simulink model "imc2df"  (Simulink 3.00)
settings: Solver=ode45  SolverMode=SingleTasking  StartTime=0.0  StopTime=10  FixedStep=st_size  MaxStep=st_size  RelTol=1e-5  AbsTol=1e-6
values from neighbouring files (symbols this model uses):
  d_through_p = get(MAIN_MENU(19),'Value')    [cback.m]    (also in imcmenu.m = 0)
  Disturb = Setpoint    [mimo_MSF1DF_sim.m]    (also in mimo_MSF2DF_sim.m)
  Satlb = temp1    [cback.m]    (also in imcmenu.m = str2num(satlbs))
  Satub = temp1    [cback.m]    (also in imcmenu.m = str2num(satubs))
  Setpoint = zeros(1,n)    [mimo_MSF1DF_sim.m]    (also in mimo_MSF2DF_sim.m)
undefined symbols (not defined in the file or in its folder): denCs, denCs2, denMs, denPd, denPs, numCs, numCs2, numMs, numPd, numPs, Qdden, Qdnum
libraries: MIMO_lib x2

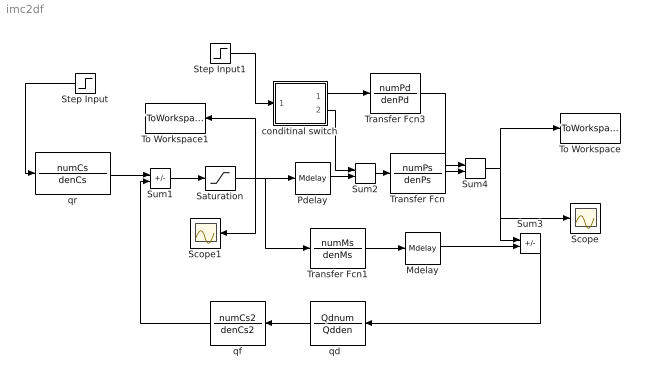
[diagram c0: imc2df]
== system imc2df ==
  Mdelay : MIMO_lib/Mdelay  Mdelay=Mdelay
  Pdelay : MIMO_lib/Mdelay  Mdelay=Pdelay
  Saturation : Saturate  UpperLimit=Satub  LowerLimit=Satlb
  Scope : Scope
  Scope1 : Scope
  Step Input : Step  Orientation=left  Time=0  Before=0  After=Setpoint  SampleTime=0
  Step Input1 : Step  Time=0  Before=0  After=Disturb  SampleTime=0
  Sum1 : Sum  Inputs=+-  SaturateOnIntegerOverflow=on
  Sum2 : Sum  Inputs=++  SaturateOnIntegerOverflow=on
  Sum3 : Sum  Inputs=+-  SaturateOnIntegerOverflow=on
  Sum4 : Sum  Inputs=++  SaturateOnIntegerOverflow=on
  To Workspace : ToWorkspace  VariableName=simout  SampleTime=-1  SaveFormat=Matrix
  To Workspace1 : ToWorkspace  VariableName=effort  SampleTime=-1  SaveFormat=Matrix
  Transfer Fcn : TransferFcn  Numerator=numPs  Denominator=denPs
  Transfer Fcn1 : TransferFcn  Numerator=numMs  Denominator=denMs
  Transfer Fcn3 : TransferFcn  Numerator=numPd  Denominator=denPd
  conditinal switch : Subsystem  Description=pass input signal through out1 if condition is true.
  "qd  " : TransferFcn  Orientation=left  Numerator=Qdnum  Denominator=Qdden
  qf : TransferFcn  Orientation=left  Numerator=numCs2  Denominator=denCs2
  qr : TransferFcn  Numerator=numCs  Denominator=denCs
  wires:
  Step Input/1 -> qr/1
  qr/1 -> Sum1/1
  Transfer Fcn1/1 -> Mdelay/1
  Mdelay/1 -> Sum3/2
  Sum3/1 -> "qd  "/1
  "qd  "/1 -> qf/1
  qf/1 -> Sum1/2
  Sum1/1 -> Saturation/1
  Saturation/1 -> Pdelay/1, Scope1/1, To Workspace1/1, Transfer Fcn1/1
  Pdelay/1 -> Sum2/2
  Sum2/1 -> Transfer Fcn/1
  Transfer Fcn/1 -> Sum4/2
  Transfer Fcn3/1 -> Sum4/1
  Step Input1/1 -> conditinal switch/1(In)
  conditinal switch/1(Out2) -> Transfer Fcn3/1
  conditinal switch/2(Out1) -> Sum2/1
  Sum4/1 -> Sum3/1, To Workspace/1, Scope/1

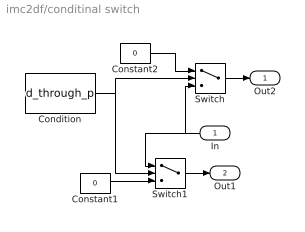
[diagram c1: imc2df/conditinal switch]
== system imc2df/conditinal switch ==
  In : Inport  Orientation=left  Port=1  PortWidth=-1  SampleTime=-1  DataType=auto
  Condition : Constant  Value=d_through_p
  Constant1 : Constant  Value=0
  Constant2 : Constant  Value=0
  Switch : Switch  Threshold=1
  Switch1 : Switch  Threshold=1
  Out2 : Outport  Port=1  InitialOutput=0
  Out1 : Outport  Port=2  InitialOutput=0
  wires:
  In/1 -> Switch/3, Switch1/1
  Condition/1 -> Switch1/2, Switch/2
  Constant1/1 -> Switch1/3
  Constant2/1 -> Switch/1
  Switch/1 -> Out2/1
  Switch1/1 -> Out1/1
